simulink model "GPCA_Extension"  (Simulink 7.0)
settings: Solver=ode45  StartTime=0.0  StopTime=inf  RelTol=1e-3
PreLoadFcn:
  | GPCA_Bus_Def
InitFcn:
  | script
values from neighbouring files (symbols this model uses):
  GOutputEvents = [0 0 0 0 0 0 0 0 0 0 0 0 0 0 0 0 0 0 0 0 0]    [script.m]
  GProgrammedDoseRate = 0    [script.m]
  GProgrammedVTBI = 0    [script.m]
undefined symbols (not defined in the file or in its folder): BarcodeReader, patientReader, y1, y2, y3, y4, y5, y6
libraries: simulink x3
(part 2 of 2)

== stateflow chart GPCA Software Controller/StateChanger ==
  state x = displayBolusInfo [function]
    (junction 152) -> (junction 154) : [infuStatus.isBolusInProgress == 1]{bolusing := 1; ml.GAlrmMsg = MSG_BOLUSGRANT; }
    (default) -> (junction 152)
    (junction 152) -> (junction 153) : [infuStatus.isBolusInProgress == 0]{ml.GAlrmMsg = MSG_BOLUSDENIED; }
  state x1 = enterinto(stateId) [function]
    (junction 88) -> (junction 89) : {x1 := stateId;}
    (default) -> (junction 88) : {O_CurrentState := stateId;}
  state x = resumeInfusion [function]
    (junction 200) -> (junction 109) : {O_InfusionInProgress := 1;  O_InfusionPaused := 0;  O_BolusRequested := 0;}
    (default) -> (junction 199)
    (junction 199) -> (junction 200) : {infusing := 1; bolusing := 0;}
  state x = warning [function]
    (junction 127) -> (junction 108) : [ErrCond == 17]{ml.GAlrmMsg = MSG_LOWRESR;}
    (junction 127) -> (junction 128) : [ErrCond == 16]{ml.GAlrmMsg = MSG_FLOWRATEVARY;}
    (junction 127) -> (junction 115) : [ErrCond == 19]{ml.GAlrmMsg = MSG_LOGERR; }
    (junction 127) -> (junction 120) : [ErrCond == 26]{ml.GAlrmMsg = MSG_DANGERAP;}
    (junction 127) -> (junction 121) : [ErrCond ==18]{ml.GAlrmMsg = MSG_PAUSELONG;}
    (junction 127) -> (junction 122) : [ErrCond==20]{ml.GAlrmMsg = MSG_LOWBATT; }
    (junction 127) -> (junction 123) : [ErrCond==21]{ml.GAlrmMsg = MSG_WRNBATTERYCHARGE;}
    (junction 127) -> (junction 125) : [ErrCond==22]{ml.GAlrmMsg = MSG_VOLTOUTRANGE;}
    (junction 127) -> (junction 126) : [ErrCond==23]{ml.GAlrmMsg = MSG_PUMPOVERHEAT;}
    (default) -> (junction 127) : {O_AlarmCond := ErrCond;}
    (junction 127) -> (junction 131) : [ErrCond==24]{ml.GAlrmMsg = MSG_DANGERENVTEMP;}
    (junction 127) -> (junction 137) : [ErrCond == 25]{ml.GAlrmMsg = MSG_DANGERHUMD;}
  state x = initInfusion [function]
    (default) -> (junction 138)
    (junction 138) -> (junction 139) : { bolusing := 0; infusing := 0; doseRate := 0; vtbi := 0;   resetInfusionInstructions();}
  state x = checkDoseRate(iRate) [function]
    (junction 188) -> (junction 173) : [iRate <= drugLibInfo.doseRateUpperHardLimit && iRate >= drugLibInfo.doseRateLowerHardLimit]
    (junction 173) -> (junction 148) : [iRate > drugLibInfo.doseRateUpperSoftLimit || iRate < drugLibInfo.doseRateLowerSoftLimit]{ x := 1;}
    (junction 188) -> (junction 157) : [iRate > drugLibInfo.doseRateUpperHardLimit || iRate < drugLibInfo.doseRateLowerHardLimit]{ x := 2;}
    (junction 173) -> (junction 91) : [iRate <= drugLibInfo.doseRateUpperSoftLimit && iRate >= drugLibInfo.doseRateLowerSoftLimit]{ x:= 0;}
    (default) -> (junction 188)
  state x = clearAlrm (alrm) [function]
    (default) -> (junction 93) : {ClearCond := alrm;}
    (junction 93) -> (junction 94) : {E_AlarmClear;}
  state x = setPatientInfo [function]
    (default) -> (junction 167)
    (junction 167) -> (junction 169) : {O_PatientInfo.patientID := patientInfo.patientID;  O_PatientInfo.patientAge := patientInfo.patientAge;  O_PatientInfo.patientGender := patientInfo.patientGender; O_PatientInfo.patientWeight := patientInfo.patientWeight;}
  state x = initPatientInfo [function]
    (junction 187) -> (junction 144) : { O_PatientInfo.patientID := 0;  O_PatientInfo.patientAge := 0;   O_PatientInfo.patientGender := 0; O_PatientInfo.patientWeight := 0;}
    (default) -> (junction 187)
  state x = setDrugLibInfo [function]
    (junction 124) -> (junction 155) : { O_DrugLibInfo.drugConcentrationTypical = drugLibInfo.drugConcentrationTypical;   O_DrugLibInfo.drugConcentrationUpperHardLimit = drugLibInfo.drugConcentrationUpperHardLimit;   O_DrugLibInfo.drugConcentrationUpperSoftLimit = drugLibInfo.drugConcentrationUpperSoftLimit;   O_DrugLibInfo.drugConcentrationLowerSoftLimit = drugLibInfo.drugConcentrationLowerSoftLimit;   O_DrugLibInfo.drugConcentrationLowerHardLimit = drugLibInfo.drugConcentrationLowerHardLimit;}
    (default) -> (junction 132)
    (junction 132) -> (junction 143) : {O_DrugLibInfo.drugID = drugLibInfo.drugID; O_DrugLibInfo.amount = drugLibInfo.amount;}
    (junction 143) -> (junction 112) : { O_DrugLibInfo.doseRateTypical = drugLibInfo.doseRateTypical; O_DrugLibInfo.doseRateUnit = drugLibInfo.doseRateUnit;   O_DrugLibInfo.doseRateUpperHardLimit = drugLibInfo.doseRateUpperHardLimit;   O_DrugLibInfo.doseRateUpperSoftLimit = drugLibInfo.doseRateUpperSoftLimit;   O_DrugLibInfo.doseRateLowerSoftLimit = drugLibInfo.doseRateLowerSoftLimit;   O_DrugLibInfo.doseRateLowerHardLimit = drugLibInfo.doseRateLowerHardLimit;}
    (junction 112) -> (junction 124) : { O_DrugLibInfo.vtbiTypical = drugLibInfo.vtbiTypical; O_DrugLibInfo.vtbiUnit = drugLibInfo.vtbiUnit;   O_DrugLibInfo.vtbiUpperHardLimit = drugLibInfo.vtbiUpperHardLimit;   O_DrugLibInfo.vtbiUpperSoftLimit = drugLibInfo.vtbiUpperSoftLimit;   O_DrugLibInfo.vtbiLowerSoftLimit = drugLibInfo.vtbiLowerSoftLimit;   O_DrugLibInfo.vtbiLowerHardLimit = drugLibInfo.vtbiLowerHardLimit;}
  state x = setLOneMsg(fcond) [function]
    (default) -> (junction 98) : {O_AlarmCond := fcond;}
    (junction 98) -> (junction 99) : [fcond==1]{ml.GAlrmMsg =MSG_OUTOFPOWER;}
    (junction 98) -> (junction 101) : [fcond==3]{ml.GAlrmMsg = MSG_CPUFAILURE;}
    (junction 98) -> (junction 102) : [fcond==4]{ml.GAlrmMsg = MSG_MEMORYCORRUPT;}
    (junction 98) -> (junction 103) : [fcond==5]{ml.GAlrmMsg = MSG_PUMPTOOHOT;}
    (junction 98) -> (junction 104) : [fcond==6]{ml.GAlrmMsg = MSG_WATCHDOGALERT;}
    (junction 98) -> (junction 100) : [fcond==2]{ml.GAlrmMsg = MSG_REALTIMECLOCK;}
  state x = alrmLevel [function]
    (junction 96) -> (junction 184) : [ErrCond == 0]{O_AlarmCond := ErrCond; x := 0;}
    (default) -> (junction 96)
    (junction 96) -> (junction 129) : [ErrCond  > 0 && ErrCond <7] {O_AlarmCond := ErrCond; x:=1;}
    (junction 96) -> (junction 90) : [ErrCond>=7 && ErrCond < 16]{O_AlarmCond := ErrCond; x:=2;}
    (junction 96) -> (junction 97) : [ErrCond>=16]{O_AlarmCond := ErrCond; x:=3;}
  state x = setLTwoMsg(fCond) [function]
    (junction 111) -> (junction 107) : [fCond==14]{ml.GAlrmMsg = MSG_PAUSETOOLONG;}
    (junction 111) -> (junction 105) : [fCond==9]{ml.GAlrmMsg = MSG_OCCULUSION;}
    (junction 111) -> (junction 110) : [fCond==15]{ml.GAlrmMsg = MSG_AIRINLINE;}
    (default) -> (junction 111) : {O_AlarmCond := fCond;}
    (junction 111) -> (junction 113) : [fCond==7]{ml.GAlrmMsg = MSG_DOOROPEN;}
    (junction 111) -> (junction 114) : [fCond==8]{ml.GAlrmMsg = MSG_EMPTYRESERVOIR;}
    (junction 111) -> (junction 116) : [fCond==10]{ml.GAlrmMsg = MSG_OVERINFUSION;}
    (junction 111) -> (junction 117) : [fCond==11]{ml.GAlrmMsg = MSG_UNDERINFUSION;}
    (junction 111) -> (junction 118) : [fCond==12]{ml.GAlrmMsg = MSG_LESSTHANKVO;}
    (junction 111) -> (junction 119) : [fCond==13]{ml.GAlrmMsg = MSG_RATEEXCEEDCAPACITY;}
  state x = bolusStatus [function]
    (default) -> (junction 134)
    (junction 134) -> (junction 135) : [infuStatus.isBolusInProgress == 1]{bolusing := 1; ml.GAlrmMsg = MSG_BOLUSGRANT;}
    (junction 134) -> (junction 136) : [infuStatus.isBolusInProgress == 0]{bolusing := 0; ml.GAlrmMsg = MSG_BOLUSDENIED;}
  state x = checkVTBI(inputVal) [function]
    (default) -> (junction 156)
    (junction 145) -> (junction 92) : [inputVal <= drugLibInfo.vtbiUpperSoftLimit && inputVal <= drugLibInfo.vtbiLowerSoftLimit]{ x := 0;}
    (junction 145) -> (junction 95) : [inputVal > drugLibInfo.vtbiUpperSoftLimit || inputVal < drugLibInfo.vtbiLowerSoftLimit]{ x := 1;}
    (junction 156) -> (junction 146) : [inputVal > drugLibInfo.vtbiUpperHardLimit || inputVal < drugLibInfo.vtbiLowerHardLimit]{ x := 2;}
    (junction 156) -> (junction 145) : [inputVal <= drugLibInfo.vtbiUpperHardLimit && inputVal >= drugLibInfo.vtbiLowerHardLimit]
  state x = calcFlowRate(iRate) [function]
    (junction 163) -> (junction 164) : {x := iRate /  drugInfo.drugConcentration;}
    (default) -> (junction 163)
  state x = checkDrugConcentration [function]
    (junction 174) -> (junction 172) : [actualCon > upperHard || actualCon < lowerHard]{x := 2;}
    (junction 174) -> (junction 178) : [actualCon <= upperHard && actualCon >= lowerHard]
    (default) -> (junction 174) : {actualCon := drugInfo.drugConcentration; upperHard := drugLibInfo.drugConcentrationUpperHardLimit; upperSoft := drugLibInfo.drugConcentrationUpperSoftLimit; lowerHard := drugLibInfo.drugConcentrationLowerHardLimit;  lowerSoft := drugLibInfo.drugConcentrationLowerSoftLimit;}
    (junction 178) -> (junction 176) : [actualCon <= upperSoft && actualCon >= lowerSoft]{x := 0;}
    (junction 178) -> (junction 177) : [actualCon > upperSoft || actualCon < lowerSoft]{x := 1;}
  state x = initDrugLib [function]
    (junction 168) -> (junction 166) : { O_DrugLibInfo.drugID := 0; O_DrugLibInfo.amount = 0; O_DrugLibInfo.diluentVolume := 0; O_DrugLibInfo.doseRateTypical := 0;   O_DrugLibInfo.doseRateUpperHardLimit := 0; O_DrugLibInfo.doseRateUpperSoftLimit := 0; O_DrugLibInfo.doseRateLowerHardLimit := 0;   O_DrugLibInfo.doseRateLowerSoftLimit := 0; O_DrugLibInfo.doseRateUnit := 0; O_DrugLibInfo.vtbiTypical := 0; O_DrugLibInfo.vtbiUpperHardLimit := 0;   O_DrugLibInfo.vtbiUpperSoftLimit := 0; O_DrugLibInfo.vtbiLowerHardLimit := 0; O_DrugLibInfo.vtbiLowerSoftLimit := 0; O_DrugLibInfo.vtbiUnit :=0;   O_DrugLibInfo.drugConcentrationTypical := 0; O_DrugLibInfo.drugConcentrationUpperHardLimit := 0; O_DrugLibInfo.drugConcentrationUpperSoftLimit := 0;   O_DrugLibInfo.drugConcentrationLowerHardLimit := 0; O_DrugLibInfo.drugConcentrationLowerSoftLimit := 0;}
    (default) -> (junction 168)
  state x = init [function]
    (junction 159) -> (junction 130) : {temp := 0; tempx := 0; infusing :=0; bolusing :=0;}
    (default) -> (junction 183)
    (junction 183) -> (junction 159) : { ClearCond := 0; O_InfusionInProgress := 0; O_InfusionPaused := 0;   O_BolusRequested := 0; O_ProgrammedVTBI := 0; O_ProgrammedFlowRate := 0; O_CurrentState := 0;   O_AlarmCond := 0;  initDrugLib(); initPatientInfo();}
  state InfusionStateMachine
    state ConfirmPowerDown
      en: enterinto(2);
      ml.GMsgConStr := MSG_POWEROFF;
    state PowerOff
      en: enterinto(1);
      ex: ml.GMsgConStr = MSG_WELCOME;
    state POST
      en: enterinto(3);
      tempx := pumpConfigData.isPOSTSuccessful ;
    state ALM_POSTFailed
      en:  ml.GMsgConStr =MSG_POSTFAIL;
      enterinto(4);
    state InfusionInSession
      state InfusionPaused
        en: enterinto(36);
        pauseInfusion();
        ml.GMsgConStr = MSG_INFUSIONPAUSED;
      state PausedStopConfirm
        en: ml.GMsgConStr = MSG_SPCHOOSE;
        enterinto(38);
      state InfusionStopped
        en: copyInfuStatus();
        stopInfusion();
        ml.GMsgConStr = MSG_INFUSIONSTOP;
        enterinto(39);
      state EmptyReservoir
        en: enterinto(40);
        ml.GAlrmMsg = MSG_EMPTYRESERVOIR;
      state CheckDrugWhileInfusing
        en: ml.GMsgConStr = MSG_CHECKTYPE
        enterinto(41);
        tempx := checkDrug();
      state ALMWrongDrug
        en: ml.GMsgConStr = MSG_WRONGDRUG;
        enterinto(42);
      state LevelTwoAlarming
        en: enterinto(44);
        setLTwoMsg(ErrCond);
      state InfusionSubMachine
        state Infusing
          en:  ml.GMsgConStr = MSG_INFUSING;
          enterinto(28);
          copyInfuStatus();
          on every(3, E_Clock):
          copyInfuStatus();
        state ChangeRate
          en: ml.GMsgConStr = MSG_CHANGEDR;
          ml.GSetConVal =temp;
          enterinto(30);
          copyInfuStatus();
          on every(3, E_Clock):
          copyInfuStatus();
        state CheckNewRate
          en: ml.GMsgConStr = MSG_CHECKDR;
          tempx = checkDoseRate(infuParameters.programmedDoseRate);
          temp = infuParameters.programmedDoseRate;
          enterinto(31);
          copyInfuStatus();
          on every(3, E_Clock):
          copyInfuStatus();
        state ALM_NewRateOutBound
          en: ml.GMsgConStr = MSG_ALRMDR ;
          enterinto(32);
          copyInfuStatus();
          on every(3, E_Clock):
          copyInfuStatus();
        state ConfirmStop
          en: ml.GMsgConStr = MSG_CONFIRMSTOP;
          enterinto(35);
          copyInfuStatus();
          on every(3, E_Clock):
          copyInfuStatus();
        state ConfirmPause
          en: ml.GMsgConStr = MSG_CONFIRMPAUSE;
          enterinto(34);
          copyInfuStatus();
          on every(3, E_Clock):
          copyInfuStatus();
        state BolusRequest
          en: enterinto(29);
        Infusing -> ConfirmPause : E_PauseInfusion
        Infusing -> ChangeRate : E_ChangeDoseRate
        ChangeRate -> Infusing : E_Cancel
        ChangeRate -> CheckNewRate : E_ConfirmDoseRate
        CheckNewRate -> ALM_NewRateOutBound : [tempx>0]
        CheckNewRate -> Infusing : [tempx==0]{setDoseRate(temp); O_ProgrammedFlowRate := calcFlowRate(temp);}
        ALM_NewRateOutBound -> Infusing : E_Cancel
        (default) -> Infusing
        ConfirmPause -> Infusing : E_Cancel
        ConfirmStop -> Infusing : E_Cancel
        (junction 149) -> Infusing : [infuStatus.isBolusInProgress == 1]{ml.GAlrmMsg = MSG_BOLUSDENIED;}
        Infusing -> (junction 149) : E_RequestBolus
        ConfirmPause -> InfusionSubMachine : E_ConfirmPauseInfusion{ml.GAlrmMsg = MSG_BLANK;}
        Infusing -> InfusionSubMachine : [infusionDone(vtbi) == 1] {ml.GAlrmMsg = MSG_BLANK;}
        Infusing -> ConfirmStop : E_StopInfusion
        ConfirmStop -> InfusionSubMachine : E_ConfirmStopInfusion{ml.GAlrmMsg = MSG_BLANK;}
        ALM_NewRateOutBound -> ChangeRate : E_ChangeDoseRate
        ChangeRate -> ChangeRate : E_Warning{warning();}
        ALM_NewRateOutBound -> ALM_NewRateOutBound : E_Warning{warning();}
        ConfirmStop -> ConfirmStop : E_Warning{warning();}
        Infusing -> Infusing : E_Warning{warning();}
        ConfirmPause -> ConfirmPause : E_Warning{warning();}
        InfusionSubMachine -> Infusing : E_Ready {startInfusion();}
        BolusRequest -> (junction 133) : {O_BolusRequested := 0;}
        (junction 133) -> Infusing : {displayBolusInfo();}
        (junction 149) -> BolusRequest : [infuStatus.isBolusInProgress == 0]{O_BolusRequested := 1;}
        Infusing -> Infusing : [infusing > 0 && bolusing > 0 && infuStatus.isBolusInProgress == 0]{bolusing :=0; ml.GAlrmMsg = MSG_STOPBOLUS;}
        InfusionSubMachine -> Infusing : E_Cancel{resumeInfusion();}
        InfusionSubMachine -> Infusing : [tempx == 0]{resumeInfusion();}
        InfusionSubMachine -> Infusing : E_ClearAlarm{clearLevel2Alarm(); resumeInfusion();}
        InfusionSubMachine -> Infusing : E_ClearAlarm{ClearCond:=13; resumeInfusion();E_AlarmClear}
        ChangeRate -> Infusing : [infusionDone(vtbi) == 1]
        ALM_NewRateOutBound -> Infusing : [infusionDone(vtbi) == 1]
        ConfirmStop -> Infusing : [infusionDone(vtbi) == 1]
        ConfirmPause -> Infusing : [infusionDone(vtbi) == 1]
        ConfirmPause -> ConfirmPause : [infusing > 0 && bolusing > 0 && infuStatus.isBolusInProgress == 0]{bolusing :=0; ml.GAlrmMsg = MSG_STOPBOLUS;}
        ConfirmStop -> ConfirmStop : [infusing > 0 && bolusing > 0 && infuStatus.isBolusInProgress == 0] {bolusing :=0; ml.GAlrmMsg = MSG_STOPBOLUS;}
        ChangeRate -> ChangeRate : [infusing > 0 && bolusing > 0 && infuStatus.isBolusInProgress == 0] {bolusing :=0; ml.GAlrmMsg = MSG_STOPBOLUS;}
        ALM_NewRateOutBound -> ALM_NewRateOutBound : [infusing > 0 && bolusing > 0 && infuStatus.isBolusInProgress == 0] {bolusing :=0; ml.GAlrmMsg = MSG_STOPBOLUS;}
      state PausedTooLong
        en: enterinto(37);
        ml.GAlrmMsg = MSG_PAUSETOOLONG;
      InfusionPaused -> LevelTwoAlarming : [alrmLevel()==2]{pauseInfusion();}
      InfusionInSession -> InfusionSubMachine : E_Ready {startInfusion();}
      InfusionStopped -> InfusionInSession : E_NewInfusion{resetInfusionInstructions(); initInfuStatus();}
      InfusionPaused -> InfusionSubMachine : E_Cancel{resumeInfusion();}
      InfusionPaused -> PausedTooLong : E_Alarm[ErrCond == 13]
      PausedTooLong -> InfusionSubMachine : E_ClearAlarm{ClearCond:=13; resumeInfusion();E_AlarmClear}
      InfusionPaused -> PausedStopConfirm : E_StopInfusion
      PausedStopConfirm -> InfusionPaused : E_Cancel
      PausedStopConfirm -> InfusionStopped : E_ConfirmStopInfusion
      EmptyReservoir -> CheckDrugWhileInfusing : E_CheckDrug
      CheckDrugWhileInfusing -> InfusionSubMachine : [tempx == 0]{resumeInfusion();}
      CheckDrugWhileInfusing -> ALMWrongDrug : [tempx > 0]
      EmptyReservoir -> InfusionStopped : E_StopInfusion
      ALMWrongDrug -> InfusionStopped : E_StopInfusion
      LevelTwoAlarming -> EmptyReservoir : [ErrCond==7]
      (default) -> InfusionSubMachine
      InfusionSubMachine -> LevelTwoAlarming : [alrmLevel()==2]{pauseInfusion();}
      LevelTwoAlarming -> InfusionStopped : E_StopInfusion{clearLevel2Alarm();}
      ALMWrongDrug -> ALMWrongDrug : E_Warning{warning();}
      PausedStopConfirm -> LevelTwoAlarming : [alrmLevel()==2]{pauseInfusion();}
      ALMWrongDrug -> CheckDrugWhileInfusing : E_CheckDrug
      LevelTwoAlarming -> LevelTwoAlarming : E_Warning{warning();}
      EmptyReservoir -> EmptyReservoir : E_Warning{warning();}
      InfusionStopped -> InfusionStopped : E_Warning{warning();}
      InfusionPaused -> InfusionPaused : E_Warning{warning();}
      PausedStopConfirm -> PausedStopConfirm : E_Warning{warning();}
      PausedTooLong -> PausedTooLong : E_Warning{warning();}
      LevelTwoAlarming -> InfusionSubMachine : E_ClearAlarm{clearLevel2Alarm(); resumeInfusion();}
      PausedTooLong -> InfusionStopped : E_StopInfusion
      InfusionSubMachine -> InfusionStopped : [infusionDone(vtbi) == 1] {ml.GAlrmMsg = MSG_BLANK;}
      Infusing -> InfusionStopped : [infusionDone(vtbi) == 1] {ml.GAlrmMsg = MSG_BLANK;}
      InfusionPaused -> Infusing : E_Cancel{resumeInfusion();}
      CheckDrugWhileInfusing -> Infusing : [tempx == 0]{resumeInfusion();}
      LevelTwoAlarming -> Infusing : E_ClearAlarm{clearLevel2Alarm(); resumeInfusion();}
      PausedTooLong -> Infusing : E_ClearAlarm{ClearCond:=13; resumeInfusion();E_AlarmClear}
      InfusionSubMachine -> InfusionStopped : E_ConfirmStopInfusion{ml.GAlrmMsg = MSG_BLANK;}
      ConfirmStop -> InfusionStopped : E_ConfirmStopInfusion{ml.GAlrmMsg = MSG_BLANK;}
      InfusionSubMachine -> InfusionPaused : E_ConfirmPauseInfusion{ml.GAlrmMsg = MSG_BLANK;}
      ConfirmPause -> InfusionPaused : E_ConfirmPauseInfusion{ml.GAlrmMsg = MSG_BLANK;}
    state Init
    state POSTDONE
      en: ml.GMsgConStr = MSG_POSTDONE;
      enterinto(45);
      tempx = 0;
    state LEVELONEALRM
      en: setLOneMsg(ErrCond);
      enterinto(43);
    state CheckDrugRoutine
      state CheckAdminSet
        en: enterinto(5);
        ml.GMsgConStr =MSG_ADMINCHECK;
        tempx := pumpConfigData.isAdminSetCheckPassed;
      state CheckPrime
        en:  enterinto(7);
        tempx = 0;
        ml.GMsgConStr = MSG_PRIME;
        tempx = pumpConfigData.isPumpPrimed;
      state ALM_WrongAdminCheck
        en: enterinto(6);
        ml.GMsgConStr = MSG_ADMINFAIL;
      state PrimeFailed
        en: enterinto(8);
        ml.GMsgConStr = MSG_PRIMEFAIL;
      state DisplayDrugInfo
        en: enterinto(9);
        tempx = 0;
        ml.GMsgConStr = MSG_DRUGINFO;
      state CheckDrug_CheckType
        en: enterinto(10);
        ml.GMsgConStr = MSG_CHECKTYPE;
        tempx := checkDrugType();
      state UnknownDrug
        en: enterinto(11);
        ml.GMsgConStr =MSG_WRONGDRUG;
      state Check_DrugUnits
        en: enterinto(12);
        ml.GMsgConStr = MSG_CHECKDU;
        tempx := checkDrugUnits();
      state IncorrectDrugUnits
        en: enterinto(13);
        ml.GMsgConStr =MSG_WRONGDU;
      state Check_Concen
        en:enterinto(14);
        ml.GMsgConStr = MSG_CHECKCON;
        tempx := checkDrugConcentration();
      state WrongConcentration
        en: enterinto(15);
        ml.GMsgConStr = MSG_WRONGCON;
      state WRN_DangerCon
        en: enterinto(16);
        ml.GMsgConStr = MSG_DANGECON;
      state DisplayPatientProfile
        en:   enterinto(18);
        ml.GMsgConStr = MSG_PATIENTINFO;
      UnknownDrug -> CheckDrug_CheckType : E_CheckDrug
      Check_Concen -> WrongConcentration : [tempx==2]
      Check_DrugUnits -> IncorrectDrugUnits : [tempx!=0]
      IncorrectDrugUnits -> CheckDrug_CheckType : E_CheckDrug
      Check_DrugUnits -> Check_Concen : [tempx==0]
      CheckDrug_CheckType -> UnknownDrug : [tempx==1]
      CheckDrug_CheckType -> Check_DrugUnits : [tempx==0]
      Check_Concen -> WRN_DangerCon : [tempx==1]
      Check_Concen -> DisplayPatientProfile : [tempx==0]{setPatientInfo();}
      WRN_DangerCon -> DisplayPatientProfile : E_ConfirmConcentration{setPatientInfo();}
      DisplayPatientProfile -> CheckDrugRoutine : E_ConfigureInfusionProgram{setDrugLibInfo();}
      ALM_WrongAdminCheck -> CheckAdminSet : E_CheckAdminSet
      CheckAdminSet -> ALM_WrongAdminCheck : [tempx==0]
      CheckAdminSet -> CheckPrime : [tempx==1]{E_Restart; }
      PrimeFailed -> CheckPrime : E_Prime
      CheckPrime -> PrimeFailed : [tempx==0]
      CheckPrime -> DisplayDrugInfo : [tempx==1]{setDrugLibInfo();}
      DisplayPatientProfile -> DisplayDrugInfo : E_Cancel
      DisplayDrugInfo -> CheckDrug_CheckType : E_CheckDrug
      ALM_WrongAdminCheck -> ALM_WrongAdminCheck : E_Warning{warning();}
      UnknownDrug -> UnknownDrug : E_Warning{warning();}
      WrongConcentration -> CheckDrug_CheckType : E_CheckDrug
      WrongConcentration -> WrongConcentration : E_Warning{warning();}
      CheckDrugRoutine -> CheckAdminSet : E_NewInfusion{resetInfusionInstructions(); initInfuStatus();}
      CheckDrugRoutine -> CheckAdminSet : E_CheckAdminSet{resetInfusionInstructions(); initInfuStatus();}
      DisplayDrugInfo -> DisplayDrugInfo : E_Warning{warning();}
      WRN_DangerCon -> WRN_DangerCon : E_Warning{warning();}
      WRN_DangerCon -> CheckDrug_CheckType : E_CheckDrug
      DisplayPatientProfile -> DisplayPatientProfile : E_Warning{warning();}
      PrimeFailed -> PrimeFailed : E_Warning{warning();}
      IncorrectDrugUnits -> IncorrectDrugUnits : E_Warning{warning();}
    state ConfigureInfusionProgram
      state ALM_VTBIOutBound
        en: enterinto(22);
        ml.GMsgConStr = MSG_ALMVTBI;
      state DisplayDoseRate
        en:  enterinto(23);
        ml.GMsgConStr = MSG_DISPLAYDR;
        tempx = 0;
        setDoseRate(drugLibInfo.doseRateTypical);
      state DisplayVTBI
        en:   enterinto(19);
        ml.GMsgConStr = MSG_VTBI;
        setVTBI(drugLibInfo.vtbiTypical);
      state ChangeVTBI
        en: enterinto(20);
        ml.GMsgConStr = MSG_CHANGEVTBI;
      state CheckVTBI
        en: enterinto(21);
        ml.GMsgConStr = MSG_CHECKVTBI;
        tempx := checkVTBI(infuParameters.programmedVTBI);
      state ChangeDoseRate
        en: enterinto(24);
        ml.GMsgConStr = MSG_CHANGEDR;
      state CheckDoseRate
        en: enterinto(25);
        ml.GMsgConStr = MSG_CHECKDR;
        tempx := checkDoseRate(infuParameters.programmedDoseRate);
      state ALM_DoseRateOutBound
        en: enterinto(26);
        ml.GMsgConStr = MSG_ALRMDR;
      state DisplaySettings
        en: enterinto(27);
        ml.GMsgConStr = MSG_DISPLAYSET;
      state ReadyToStart
        en: enterinto(48);
      state WRN_VTBIOutBound
        en: enterinto(46);
        ml.GMsgConStr = MSG_WRNVTBI;
      state WRN_DOSERATEOUTSOFTLIMITS
        en:  enterinto(47);
        ml.GMsgConStr = MSG_WRNDR;
      CheckVTBI -> ALM_VTBIOutBound : [tempx==2]
      ALM_VTBIOutBound -> ChangeVTBI : E_ChangeVTBI
      CheckVTBI -> DisplayDoseRate : [tempx==0]{setVTBI(infuParameters.programmedVTBI);}
      ChangeVTBI -> CheckVTBI : E_ConfirmVTBI
      DisplayVTBI -> ChangeVTBI : E_ChangeVTBI
      ChangeVTBI -> DisplayVTBI : E_Cancel
      DisplayVTBI -> DisplayDoseRate : E_ConfirmVTBI
      DisplayDoseRate -> ChangeDoseRate : E_ChangeDoseRate
      ChangeDoseRate -> DisplayDoseRate : E_Cancel
      ChangeDoseRate -> CheckDoseRate : E_ConfirmDoseRate
      CheckDoseRate -> ALM_DoseRateOutBound : [tempx==2]
      ALM_DoseRateOutBound -> ChangeDoseRate : E_ChangeDoseRate
      CheckDoseRate -> DisplaySettings : [tempx==0]{setDoseRate(infuParameters.programmedDoseRate);}
      DisplayDoseRate -> DisplaySettings : E_ConfirmDoseRate
      DisplaySettings -> ReadyToStart : E_StartInfusion{E_RequestToStart}
      DisplaySettings -> DisplaySettings : E_Warning{warning();}
      WRN_VTBIOutBound -> WRN_VTBIOutBound : E_Warning{warning();}
      ReadyToStart -> ReadyToStart : E_Warning{warning();}
      DisplayVTBI -> DisplayVTBI : E_Warning{warning();}
      ReadyToStart -> DisplaySettings : E_NotReady{ml.GAlrmMsg = MSG_NOTREADY;}
      DisplaySettings -> DisplayVTBI : E_ConfigureInfusionProgram
      ChangeDoseRate -> ChangeDoseRate : E_Warning{warning();}
      ReadyToStart -> ConfigureInfusionProgram : E_Ready {startInfusion();}
      CheckVTBI -> WRN_VTBIOutBound : [tempx==1]
      WRN_VTBIOutBound -> DisplayDoseRate : E_ConfirmVTBI{setVTBI(infuParameters.programmedVTBI);}
      WRN_VTBIOutBound -> ChangeVTBI : E_ChangeVTBI
      ConfigureInfusionProgram -> DisplayVTBI : E_ConfigureInfusionProgram{setDrugLibInfo();}
      WRN_DOSERATEOUTSOFTLIMITS -> DisplaySettings : E_ConfirmDoseRate{setDoseRate(infuParameters.programmedDoseRate);}
      CheckDoseRate -> WRN_DOSERATEOUTSOFTLIMITS : [tempx==1]
      DisplayDoseRate -> DisplayDoseRate : E_Warning{warning();}
      ALM_DoseRateOutBound -> ALM_DoseRateOutBound : E_Warning{warning();}
      ALM_VTBIOutBound -> ALM_VTBIOutBound : E_Warning{warning();}
      ChangeVTBI -> ChangeVTBI : E_Warning{warning();}
      WRN_DOSERATEOUTSOFTLIMITS -> ChangeDoseRate : E_ChangeDoseRate
    Init -> PowerOff
    ALM_POSTFailed -> PowerOff : E_PowerButton
    PowerOff -> POST : E_PowerButton{init(); ml.GMsgConStr = MSG_POST;}
    ConfirmPowerDown -> CheckDrugRoutine : E_Cancel[tempx==1]
    InfusionInSession -> ConfirmPowerDown : E_PowerButton{tempx=3;}
    POSTDONE -> POSTDONE : E_Warning{warning();}
    ConfirmPowerDown -> PowerOff : E_ConfirmPowerDown{O_AlarmCond := 0; ml.GAlrmMsg := MSG_BLANK;}
    ConfirmPowerDown -> ConfigureInfusionProgram : E_Cancel[tempx==2]
    ConfigureInfusionProgram -> ConfirmPowerDown : E_PowerButton{tempx=2;}
    ConfirmPowerDown -> InfusionInSession : E_Cancel[tempx==3]
    InfusionInSession -> LEVELONEALRM : [alrmLevel()==1]{resetInfusionInstructions();}
    InfusionStopped -> CheckAdminSet : E_NewInfusion{resetInfusionInstructions(); initInfuStatus();}
    POSTDONE -> CheckAdminSet : E_CheckAdminSet{resetInfusionInstructions(); initInfuStatus();}
    ConfirmPowerDown -> ConfirmPowerDown : E_Warning{warning();}
    ALM_POSTFailed -> ALM_POSTFailed : E_Warning{warning();}
    POST -> ALM_POSTFailed : [tempx==0]
    CheckDrugRoutine -> LEVELONEALRM : [alrmLevel()==1]
    (default) -> Init
    ConfigureInfusionProgram -> LEVELONEALRM : [alrmLevel()==1]
    LEVELONEALRM -> PowerOff : E_PowerButton {O_AlarmCond := 0; ml.GAlrmMsg := MSG_BLANK;}
    POSTDONE -> ConfirmPowerDown : E_PowerButton{tempx=4;}
    ConfirmPowerDown -> POSTDONE : E_Cancel[tempx==4]
    POST -> POSTDONE : [tempx==1]
    POSTDONE -> CheckDrugRoutine : E_CheckAdminSet{resetInfusionInstructions(); initInfuStatus();}
    DisplayPatientProfile -> DisplayVTBI : E_ConfigureInfusionProgram{setDrugLibInfo();}
    ConfigureInfusionProgram -> InfusionInSession : E_Ready {startInfusion();}
    ReadyToStart -> Infusing : E_Ready {startInfusion();}
    InfusionInSession -> CheckDrugRoutine : E_NewInfusion{resetInfusionInstructions(); initInfuStatus();}
    CheckDrugRoutine -> ConfirmPowerDown : E_PowerButton{tempx=1;}
    CheckDrugRoutine -> ConfigureInfusionProgram : E_ConfigureInfusionProgram{setDrugLibInfo();}
  state x = infusionDone(expectedVolume) [function]
    (default) -> (junction 106) : {x:=0;}
    (junction 106) -> (junction 141) : [infuStatus.totalVolumeInfused < expectedVolume]{x := 0;}
    (junction 106) -> (junction 142) : [infuStatus.totalVolumeInfused >= expectedVolume]{x := 1;}
  state x = clearLevel2Alarm [function]
    (junction 185) -> (junction 186) : {ml.GAlrmMsg = MSG_BLANK; E_AlarmClear;}
    (default) -> (junction 185)
  state x = checkDrugType [function]
    (junction 181) -> (junction 175) : [drugInfo.drugDoseAmount == drugLibInfo.amount]{x := 0;}
    (junction 181) -> (junction 171) : [drugInfo.drugDoseAmount != drugLibInfo.amount]{x := 1;}
    (default) -> (junction 182)
    (junction 182) -> (junction 147) : [drugInfo.drugID != drugLibInfo.drugID]{x:=1;}
    (junction 182) -> (junction 181) : [drugInfo.drugID == drugLibInfo.drugID]
  state x = checkDrug [function]
    (junction 162) -> (junction 161) : [flag == 1]{x := 1;}
    (default) -> (junction 162) : {flag := checkDrugType();}
    (junction 192) -> (junction 140) : [flag == 1]{x := 1;}
    (junction 192) -> (junction 189) : [flag == 0]{flag:= checkDrugConcentration();}
    (junction 189) -> (junction 191) : [flag == 0]{x := 0;}
    (junction 189) -> (junction 190) : [flag > 0]{x := 1;}
    (junction 162) -> (junction 192) : [flag == 0]{flag := checkDrugUnits();}
  state x = checkDrugUnits [function]
    (junction 150) -> (junction 158) : [drugInfo.drugVolumeUnit == drugLibInfo.vtbiUnit]{ x:= 0;}
    (default) -> (junction 170)
    (junction 150) -> (junction 160) : [drugInfo.drugVolumeUnit != drugLibInfo.vtbiUnit]{x := 1;}
    (junction 170) -> (junction 150) : [drugInfo.drugDoseUnit == drugLibInfo.doseRateUnit]
    (junction 170) -> (junction 151) : [drugInfo.drugDoseUnit != drugLibInfo.doseRateUnit]{x := 1;}
  state x = stopInfusion [function]
    (junction 194) -> (junction 193) : {O_ProgrammedVTBI := 0;  O_ProgrammedFlowRate := 0;}
    (junction 209) -> (junction 194) : {O_InfusionInProgress := 0;  O_InfusionPaused := 0;  O_BolusRequested := 0;}
    (default) -> (junction 208)
    (junction 208) -> (junction 209) : {infusing := 0; bolusing := 0;}
  state x = setVTBI(iVTBI) [function]
    (default) -> (junction 195)
    (junction 195) -> (junction 196) : {vtbi := iVTBI;}
  state x = setDoseRate(iRate) [function]
    (default) -> (junction 197)
    (junction 197) -> (junction 198) : {doseRate := iRate;}
  state x = startInfusion [function]
    (default) -> (junction 201)
    (junction 201) -> (junction 202) : {O_ProgrammedFlowRate := calcFlowRate(doseRate);  O_ProgrammedVTBI := vtbi;}
    (junction 202) -> (junction 203) : {O_InfusionInProgress := 1;  O_InfusionPaused := 0;  O_BolusRequested := 0;}
    (junction 203) -> (junction 204) : {infusing := 1; bolusing := 0;}
  state x = pauseInfusion [function]
    (default) -> (junction 205)
    (junction 205) -> (junction 206) : {infusing := 0; bolusing := 0;}
    (junction 206) -> (junction 207) : {O_InfusionInProgress := 1;  O_InfusionPaused := 1;  O_BolusRequested := 0;}
  state x = resetInfusionInstructions [function]
    (junction 211) -> (junction 210) : {stopInfusion();}
    (default) -> (junction 211)
  state x = copyInfuStatus [function]
    (default) -> (junction 212)
    (junction 212) -> (junction 213) : {O_InfuStatus.isBolusInProgress := infuStatus.isBolusInProgress;  O_InfuStatus.totalVolumeInfused := infuStatus.totalVolumeInfused;  O_InfuStatus.remainingVolumeInReservoir := infuStatus.remainingVolumeInReservoir;}
  state x = initInfuStatus [function]
    (default) -> (junction 214)
    (junction 214) -> (junction 215) : {O_InfuStatus.isBolusInProgress := 0;  O_InfuStatus.totalVolumeInfused := 0;  O_InfuStatus.remainingVolumeInReservoir := infuStatus.remainingVolumeInReservoir;}
  state x = outputInfuStatus(a,b,c) [function]
    (default) -> (junction 216)
    (junction 216) -> (junction 217) : {O_InfuStatus.isBolusInProgress := a;  O_InfuStatus.totalVolumeInfused := b;  O_InfuStatus.remainingVolumeInReservoir := c;}

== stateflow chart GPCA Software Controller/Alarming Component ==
  state AlarmingMachine
    state WRN [parallel]
      state HumidityCheck
      state BatteryChargingCheck
      state LowBatteryCheck
      state LoggingCheck
      state InfusionPausedDurationCheck
      state EndState
      state WNStart
        en: WnCond = 0;
      state LowReservoirCheck
      state VoltageCheck
      state FlowRateStabilityCheck
      state HoldOn
      state PumpTempCheck
      state EnvTempCheck
      state APErrCheck
      (junction 797) -> (junction 796)
      BatteryChargingCheck -> VoltageCheck : [hardwareSenData.isBatteryUnableToCharge == 0]{clearWarning(21);}
      (junction 798) -> (junction 797)
      LowBatteryCheck -> BatteryChargingCheck : [hardwareSenData.isBatteryLow ==0]{clearWarning(20);}
      LoggingCheck -> LowBatteryCheck : [hardwareSenData.isLoggingFailed == 0]{clearWarning(19);}
      (junction 813) -> LowReservoirCheck : {WnCond := 16; send(E_WarningAlarm, Controller);}
      LowReservoirCheck -> (junction 814) : [infuSenData.isReservoirLow > 0 && infusionInProgress > 0 ]
      (junction 818) -> VoltageCheck : {WnCond := 21; send(E_WarningAlarm, Controller);}
      LowReservoirCheck -> (junction 791) : E_ResetThree
      InfusionPausedDurationCheck -> (junction 792) : E_ResetThree
      LowReservoirCheck -> InfusionPausedDurationCheck : [infuSenData.isReservoirLow == 0 || infusionInProgress == 0 ]{clearWarning(17);}
      LoggingCheck -> (junction 793) : E_ResetThree
      LowBatteryCheck -> (junction 795) : E_ResetThree
      BatteryChargingCheck -> (junction 796) : E_ResetThree
      EndState -> WNStart : E_Clock{send(E_DoneThree, Controller);}
      (junction 823) -> (junction 821)
      VoltageCheck -> (junction 758) : [hardwareSenData.isSupplyVoltageOutOfRange > 0]
      (default) -> WNStart
      WNStart -> HoldOn : E_ResetThree
      HoldOn -> FlowRateStabilityCheck : E_Clock{WnCond := 0;}
      (junction 819) -> EnvTempCheck : {WnCond := 23; send(E_WarningAlarm, Controller);}
      PumpTempCheck -> (junction 819) : [hardwareSenData.isPumpOverheated > 0]
      (junction 816) -> LowBatteryCheck : {WnCond := 19; send(E_WarningAlarm, Controller);}
      VoltageCheck -> (junction 797) : E_ResetThree
      PumpTempCheck -> (junction 798) : E_ResetThree
      (junction 814) -> InfusionPausedDurationCheck : {WnCond := 17; send(E_WarningAlarm, Controller);}
      InfusionPausedDurationCheck -> LoggingCheck : [infuSenData.isInfusionPausedLong == 0 || infusionInProgress == 0 || infusionPaused == 0]{clearWarning(18);}
      (junction 758) -> PumpTempCheck : {WnCond := 22; send(E_WarningAlarm, Controller);}
      (junction 822) -> APErrCheck : {WnCond := 25; send(E_WarningAlarm, Controller);}
      (junction 781) -> WNStart : E_Clock{send(E_DoneThree, Controller);}
      BatteryChargingCheck -> (junction 818) : [hardwareSenData.isBatteryUnableToCharge > 0]
      (junction 817) -> BatteryChargingCheck : {WnCond := 20; send(E_WarningAlarm, Controller);}
      LowBatteryCheck -> (junction 817) : [hardwareSenData.isBatteryLow > 0]
      FlowRateStabilityCheck -> (junction 794) : E_ResetThree
      FlowRateStabilityCheck -> LowReservoirCheck : [infuSenData.isFlowRateNotStable == 0 || infusionInProgress == 0 || infusionPaused == 0]{clearWarning(16);}
      FlowRateStabilityCheck -> (junction 813) : [infuSenData.isFlowRateNotStable > 0 && infusionInProgress > 0 && infusionPaused == 0]
      (junction 794) -> HoldOn
      (junction 791) -> (junction 794)
      (junction 792) -> (junction 791)
      (junction 793) -> (junction 792)
      (junction 795) -> (junction 793)
      (junction 796) -> (junction 795)
      InfusionPausedDurationCheck -> (junction 815) : [infuSenData.isInfusionPausedLong > 0 && infusionInProgress>0 && infusionPaused == 1]
      (junction 815) -> LoggingCheck : {WnCond := 18; send(E_WarningAlarm, Controller);}
      LoggingCheck -> (junction 816) : [hardwareSenData.isLoggingFailed > 0]
      EnvTempCheck -> (junction 821) : E_ResetThree
      EnvTempCheck -> (junction 820) : [envSenData.isTemperatureOutOfRange > 0]
      (junction 820) -> HumidityCheck : {WnCond := 24; send(E_WarningAlarm, Controller);}
      (junction 821) -> (junction 798)
      HumidityCheck -> (junction 823) : E_ResetThree
      HumidityCheck -> (junction 822) : [envSenData.isHumidityOutOfRange > 0]
      APErrCheck -> (junction 781) : [envSenData.isAirPressureOutOfRange ==0]{clearWarning(26);}
      APErrCheck -> (junction 824) : E_ResetThree
      HumidityCheck -> APErrCheck : [envSenData.isHumidityOutOfRange == 0]{clearWarning(25);}
      (junction 824) -> (junction 823)
      VoltageCheck -> PumpTempCheck : [hardwareSenData.isSupplyVoltageOutOfRange == 0]{clearWarning(22);}
      PumpTempCheck -> EnvTempCheck : [hardwareSenData.isPumpOverheated == 0]{clearWarning(23);}
      EnvTempCheck -> HumidityCheck : [envSenData.isTemperatureOutOfRange == 0]{clearWarning(24);}
      APErrCheck -> (junction 825) : [envSenData.isAirPressureOutOfRange > 0]
      (junction 825) -> EndState : {WnCond := 26; send(E_WarningAlarm, Controller);}
    state Controller [parallel]
      state SinkTWOCheckOne
      state START
        en: initiate();
      state CheckLOne
        en:  initiate();
      state CheckWRN
      state SinkOne
      state SinkTWO
      state CheckLTwo
      CheckWRN -> CheckLOne : E_DoneThree{send(E_ResetOne, LOne);}
      SinkOne -> CheckLOne : E_Restart{send(E_ResetOne, LOne);}
      CheckLOne -> SinkOne : E_LevelOneAlarm{ErrCond:=LOneCond;}
      START -> CheckLOne : E_Restart{send(E_ResetOne, LOne);}
      (default) -> START
      CheckWRN -> CheckWRN : E_WarningAlarm{ErrCond:=WnCond; E_Warning}
      CheckLTwo -> CheckWRN : E_DoneTwo{send(E_ResetThree, WRN);}
      SinkTWOCheckOne -> SinkTWO : E_DoneOne
      CheckLTwo -> SinkTWO : E_LevelTwoAlarm{ErrCond:=LTwoCond;}
      SinkTWO -> SinkTWOCheckOne : [LTwoCond>0]{send(E_ResetOne, LOne);}
      CheckLOne -> CheckLTwo : E_DoneOne{send(E_ResetTwo, LTwo);}
      CheckLTwo -> CheckLOne : E_Restart{send(E_ResetOne, LOne);}
      CheckWRN -> CheckLOne : E_Restart{send(E_ResetOne, LOne);}
      SinkTWO -> CheckLOne : E_Restart|E_AlarmClear{ErrCond := 0; send(E_ResetOne, LOne);}
      SinkTWO -> CheckLOne : E_Clock[LTwoCond==0]{ErrCond := 0; send(E_ResetOne, LOne);}
      SinkTWOCheckOne -> CheckLOne : E_Restart|E_AlarmClear{ErrCond := LOneCond; send(E_ResetOne, LOne);}
      SinkTWOCheckOne -> SinkOne : E_LevelOneAlarm{ErrCond:=LOneCond;}
    state LTwo [parallel]
      state Hold
      state Sink24
        en: LTwoCond = 10;
        send(E_LevelTwoAlarm, Controller);
      state Sink26
        en: LTwoCond=12;
        send(E_LevelTwoAlarm, Controller);
      state RateOverPumpCapacityCheck
      state LowInfusionRateCheck
      state RateLessThanKVOCheck
      state Sink25
        en: LTwoCond = 11;
        send(E_LevelTwoAlarm, Controller);
      state OcculusionCheck
      state Sink23
        en: LTwoCond = 9;
        send(E_LevelTwoAlarm, Controller);
      state HighInfusionRateCheck
      state Normal
        en: LTwoCond =0;
      state DoorOpenCheck
      state Sink22
        en: LTwoCond = 8;
        send(E_LevelTwoAlarm, Controller);
      state ReservoirEmptyCheck
      state Sink21
        en: LTwoCond=7;
        send(E_LevelTwoAlarm, Controller);
      state InfusionPauseDurationCheck
      state Sink27
        en: LTwoCond=13;
        send(E_LevelTwoAlarm, Controller);
      state AirInLineCheck
      state Sink29
        en: LTwoCond=15;
        send(E_LevelTwoAlarm, Controller);
      state Sink28
        en: LTwoCond=14;
        send(E_LevelTwoAlarm, Controller);
      AirInLineCheck -> Sink29 : [infuSenData.isAirInLineDetected > 0 && infusionInProgress > 0]
      InfusionPauseDurationCheck -> AirInLineCheck : [infuSenData.isInfusionPausedTooLong == 0  || infusionInProgress == 0 || infusionPaused == 0]
      InfusionPauseDurationCheck -> Sink28 : [infuSenData.isInfusionPausedTooLong > 0  && infusionInProgress > 0 && infusionPaused == 1]
      Sink29 -> (junction 773) : [infuSenData.isAirInLineDetected == 0 || infusionInProgress == 0]
      Sink29 -> (junction 772) : E_ResetTwo
      Sink28 -> (junction 774) : [infuSenData.isInfusionPausedTooLong == 0  || infusionInProgress == 0 || infusionPaused == 0]
      Sink28 -> (junction 775) : E_ResetTwo
      (junction 760) -> DoorOpenCheck
      (junction 773) -> (junction 774)
      AirInLineCheck -> (junction 761) : E_ResetTwo
      InfusionPauseDurationCheck -> (junction 762) : E_ResetTwo
      RateOverPumpCapacityCheck -> InfusionPauseDurationCheck : [infuSenData.isFlowRateOverPumpCapacity == 0 || infusionInProgress == 0]
      Sink27 -> (junction 776) : [infuSenData.isFlowRateOverPumpCapacity == 0 || infusionInProgress == 0]
      RateOverPumpCapacityCheck -> Sink27 : [infuSenData.isFlowRateOverPumpCapacity > 0 && infusionInProgress > 0 ]
      RateOverPumpCapacityCheck -> (junction 812) : E_ResetTwo
      Sink27 -> (junction 777) : E_ResetTwo
      RateLessThanKVOCheck -> RateOverPumpCapacityCheck : [infuSenData.isInfusionRateLessThanKVO == 0 || infusionInProgress == 0]
      Sink26 -> (junction 779) : E_ResetTwo
      RateLessThanKVOCheck -> (junction 811) : E_ResetTwo
      RateLessThanKVOCheck -> Sink26 : [infuSenData.isInfusionRateLessThanKVO > 0 && infusionInProgress > 0]
      Sink26 -> (junction 778) : [infuSenData.isInfusionRateLessThanKVO == 0 || infusionInProgress == 0]
      LowInfusionRateCheck -> RateLessThanKVOCheck : [infuSenData.isInfusionRateTooLow == 0 || infusionInProgress == 0 || infusionPaused > 0]
      Sink25 -> (junction 780) : [infuSenData.isInfusionRateTooLow == 0 || infusionInProgress == 0 || infusionPaused > 0]
      LowInfusionRateCheck -> (junction 810) : E_ResetTwo
      LowInfusionRateCheck -> Sink25 : [infuSenData.isInfusionRateTooLow > 0 && infusionInProgress > 0 && infusionPaused == 0]
      Sink25 -> (junction 769) : E_ResetTwo
      HighInfusionRateCheck -> LowInfusionRateCheck : [infuSenData.isInfusionRateTooHigh == 0 || infusionInProgress == 0 || infusionPaused > 0]
      HighInfusionRateCheck -> Sink24 : [infuSenData.isInfusionRateTooHigh > 0 && infusionInProgress > 0 && infusionPaused == 0]
      OcculusionCheck -> HighInfusionRateCheck : [infuSenData.isOcclusionDetected == 0 || infusionInProgress == 0]
      OcculusionCheck -> Sink23 : [infuSenData.isOcclusionDetected > 0 && infusionInProgress > 0]
      Sink24 -> (junction 756) : E_ResetTwo
      Sink24 -> (junction 757) : [infuSenData.isInfusionRateTooHigh == 0 || infusionInProgress == 0 || infusionPaused > 0]
      Sink23 -> (junction 770) : [infuSenData.isOcclusionDetected == 0 || infusionInProgress == 0]
      Sink23 -> (junction 771) : E_ResetTwo
      ReservoirEmptyCheck -> OcculusionCheck : [infuSenData.isReservoirEmpty == 0 || infusionInProgress == 0]
      ReservoirEmptyCheck -> Sink22 : [infuSenData.isReservoirEmpty > 0 && infusionInProgress > 0]
      ReservoirEmptyCheck -> (junction 807) : E_ResetTwo
      HighInfusionRateCheck -> (junction 809) : E_ResetTwo
      OcculusionCheck -> (junction 808) : E_ResetTwo
      Sink22 -> (junction 766) : [infuSenData.isReservoirEmpty == 0 || infusionInProgress == 0]
      Sink22 -> (junction 767) : E_ResetTwo
      Sink21 -> (junction 764) : [hardwareSenData.isReservoirDoorOpen == 0 || infusionInProgress == 0]
      Sink21 -> (junction 763) : E_ResetTwo
      DoorOpenCheck -> Sink21 : [hardwareSenData.isReservoirDoorOpen > 0 && infusionInProgress > 0]
      DoorOpenCheck -> ReservoirEmptyCheck : [hardwareSenData.isReservoirDoorOpen == 0 || infusionInProgress == 0]
      DoorOpenCheck -> (junction 806) : E_ResetTwo
      (junction 772) -> (junction 775)
      (junction 757) -> (junction 770)
      Hold -> DoorOpenCheck : E_Clock{LTwoCond=0;}
      (junction 756) -> (junction 771)
      (junction 775) -> (junction 777)
      (default) -> Normal
      Normal -> Hold : E_ResetTwo
      (junction 806) -> Hold
      (junction 808) -> (junction 807)
      (junction 809) -> (junction 808)
      (junction 807) -> (junction 806)
      (junction 812) -> (junction 811)
      (junction 811) -> (junction 810)
      (junction 810) -> (junction 809)
      (junction 774) -> (junction 776)
      (junction 761) -> (junction 762)
      (junction 762) -> (junction 812)
      (junction 780) -> (junction 757)
      (junction 769) -> (junction 756)
      (junction 770) -> (junction 766)
      (junction 771) -> (junction 767)
      (junction 766) -> (junction 764)
      (junction 767) -> (junction 763)
      (junction 768) -> DoorOpenCheck : E_Clock
      (junction 764) -> (junction 768)
      (junction 763) -> (junction 760)
      (junction 785) -> Normal : {send(E_DoneTwo, Controller);}
      AirInLineCheck -> (junction 785) : [infuSenData.isAirInLineDetected == 0 || infusionInProgress == 0]
      (junction 776) -> (junction 778)
      (junction 777) -> (junction 779)
      (junction 778) -> (junction 780)
      (junction 779) -> (junction 769)
    state LOne [parallel]
      state HOLD
      state WatchdogCheck
      state MemoryCheck
      state CPUCheck
      state RTCCheck
      state Normal
      state PumpTempCheck
      state L1Sink
      state BatteryDepletionCheck
      (junction 802) -> (junction 800)
      WatchdogCheck -> L1Sink : [hardwareSenData.isWatchDogInterruptDetected > 0]{LOneCond:=6; send(E_LevelOneAlarm, Controller);}
      PumpTempCheck -> WatchdogCheck : [hardwareSenData.isPumpTooHot == 0]
      Normal -> HOLD : E_ResetOne
      WatchdogCheck -> (junction 805) : [hardwareSenData.isWatchDogInterruptDetected==0]{send(E_DoneOne, Controller);}
      WatchdogCheck -> (junction 786) : E_ResetOne
      (default) -> Normal
      L1Sink -> HOLD : E_ResetOne
      PumpTempCheck -> L1Sink : [hardwareSenData.isPumpTooHot >0]{LOneCond:=5; send(E_LevelOneAlarm, Controller);}
      MemoryCheck -> PumpTempCheck : [hardwareSenData.isMemoryCorrupted == 0]
      MemoryCheck -> L1Sink : [hardwareSenData.isMemoryCorrupted > 0]{LOneCond:=4; send(E_LevelOneAlarm, Controller);}
      CPUCheck -> MemoryCheck : [hardwareSenData.isCPUInError == 0]
      CPUCheck -> L1Sink : [hardwareSenData.isCPUInError > 0]{LOneCond := 3; send(E_LevelOneAlarm, Controller);}
      RTCCheck -> CPUCheck : [hardwareSenData.isRTCInError > 0 == 0]
      RTCCheck -> L1Sink : [hardwareSenData.isRTCInError > 0> 0]{LOneCond:=2; send(E_LevelOneAlarm, Controller);}
      BatteryDepletionCheck -> RTCCheck : [hardwareSenData.isBatteryDepleted == 0]
      BatteryDepletionCheck -> L1Sink : [hardwareSenData.isBatteryDepleted > 0]{LOneCond:=1; send(E_LevelOneAlarm, Controller);}
      MemoryCheck -> (junction 803) : E_ResetOne
      PumpTempCheck -> (junction 804) : E_ResetOne
      CPUCheck -> (junction 802) : E_ResetOne
      RTCCheck -> (junction 800) : E_ResetOne
      BatteryDepletionCheck -> (junction 799) : E_ResetOne
      (junction 799) -> HOLD
      HOLD -> BatteryDepletionCheck : E_Clock{LOneCond=0;}
      (junction 786) -> (junction 804)
      (junction 805) -> Normal : E_Clock
      (junction 804) -> (junction 803)
      (junction 800) -> (junction 799)
      (junction 803) -> (junction 802)
    state CheckReady [parallel]
      state Normal
      state s1
      state Checking
        en: temp := isPumpReady();
      state s2
      s2 -> Normal : E_Restart
      s2 -> s2 : E_Clock{E_NotReady}
      s1 -> Normal : E_Restart
      s1 -> s1 : E_Clock[infusionInProgress == 0]{E_Ready}
      Checking -> Normal : E_Restart
      s2 -> Checking : E_RequestToStart
      s1 -> Normal : E_Clock[infusionInProgress == 1]
      s1 -> Checking : E_RequestToStart
      (default) -> Normal
      Normal -> Checking : E_RequestToStart
      Checking -> s2 : [temp == 0]
      Checking -> s1 : [temp > 0]
    (default) -> Controller
  state x = clearWarning(cond) [function]
    (junction 784) -> (junction 783) : [ErrCond != cond]{x:=0;}
    (junction 784) -> (junction 782) : [ErrCond == cond]{ml.GAlrmMsg = MSG_BLANK; ErrCond := 0;}
    (default) -> (junction 784)
  state x = isPumpReady [function]
    (junction 765) -> (junction 787) : [infuSenData.isReservoirEmpty > 0]{ x := 0;}
    (junction 759) -> (junction 789) : [hardwareSenData.isReservoirDoorOpen > 0] {x := 0;}
    (junction 765) -> (junction 759) : [infuSenData.isReservoirEmpty == 0]
    (default) -> (junction 765)
    (junction 759) -> (junction 788) : [hardwareSenData.isReservoirDoorOpen == 0]
    (junction 788) -> (junction 801) : [infuSenData.isFlowRateOverPumpCapacity > 0]{x := 0;}
    (junction 788) -> (junction 790) : [infuSenData.isFlowRateOverPumpCapacity == 0]{x := 1;}
  state x = initiate [function]
    (default) -> (junction 755) : {LOneCond := 0; LTwoCond := 0; WnCond := 0; ErrCond := 0; x:=0;}
  (default) -> AlarmingMachine

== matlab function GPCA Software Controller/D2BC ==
function y = d_to_b(u)
% This block supports the Embedded MATLAB subset.
% See the help menu for details. 

y = false;

if (u == 0)
    y = false;
else 
     y = true;
end;
